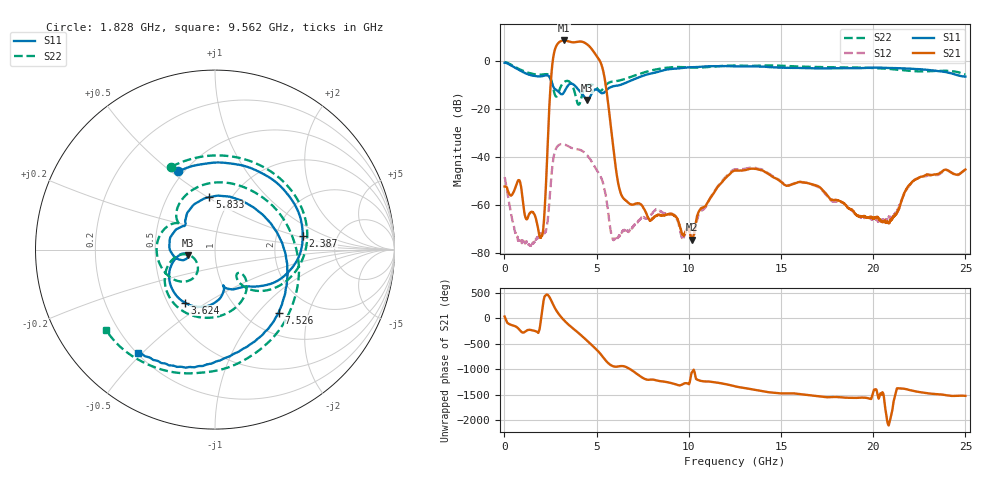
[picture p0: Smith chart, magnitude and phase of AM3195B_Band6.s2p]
!Agilent Technologies,E8364B,MY43040894,A.07.50.67
!Agilent E8364B: A.07.50.67
!Date: Wednesday, July 07, 2021 13:18:51
!Correction: S11(Full 2 Port(1,2))
!S21(Full 2 Port(1,2))
!S12(Full 2 Port(1,2))
!S22(Full 2 Port(1,2))
!S2P File: Measurements: S11, S21, S12, S22:
# Hz S  dB  R 50
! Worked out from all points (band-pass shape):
!   8001 points, 10 MHz to 25 GHz, reference 50 ohm
!   highest |S21| = 8.68 dB at 3.227 GHz (marker M1); lowest = -74.6 dB at 10.18 GHz (marker M2)
!   |S21| within 3 dB of the highest: 2.773 GHz to 4.672 GHz (1.899 GHz wide, 51 % of centre)
!   lowest |S11| = -16.2 dB at 4.489 GHz (marker M3), VSWR 1.37, Z = 36.8 - j2.45 ohm
!   |S11| at or under -10 dB: 2.614 GHz to 3.463 GHz (848.7 MHz wide, 27.9 % of centre); 3.792 GHz to 6.231 GHz (2.439 GHz wide, 48.7 % of centre)
!   |S22| runs from -18.2 to -0.3 dB; largest |S21 - S12| = 2.7
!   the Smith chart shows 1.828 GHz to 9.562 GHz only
!   S11 on the Smith chart (normalised r, x): 1.828 GHz: 0.47, +0.53; 2.387 GHz: 2.82, +0.58; 3.624 GHz: 0.61, -0.41; 5.833 GHz: 0.80, +0.51; 7.526 GHz: 1.39, -1.30; 9.562 GHz: 0.20, -0.48
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1e7  -0.62 -8.4  -52.36 38.5  -48.41 -7.3  -0.34 -9.1
1.828022e9  -6.34 115.3  -70.14 77.2  -73.52 154.5  -5.64 117.8
2.387174e9  -6.11 9.1  -26.60 90.3  -63.31 -63.2  -5.63 10.8
2.799509e9  -11.96 -57.7  6.15 165.7  -36.50 0.5  -14.78 -48.1
2.968191e9  -13.03 -74.1  7.94 76.5  -34.93 -86.6  -12.28 -44.6
3.227462e9  -13.03 -77.0  8.68 -33.6  -34.73 166.3  -8.79 -81.2
3.405516e9  -10.61 -90.0  8.46 -98.2  -35.29 103.9  -8.22 -110.6
3.624179e9  -9.37 -119.9  7.99 -168.2  -36.18 36.5  -9.40 -145.2
3.930306e9  -11.13 -155.4  8.07 100.9  -36.77 -50.2  -16.82 -167.3
4.177082e9  -13.29 -168.9  8.19 22.7  -37.30 -123.5  -15.03 -126.9
4.489458e9  -16.21 -167.9  7.04 -80.7  -39.32 141.1  -10.17 -158.3
4.726862e9  -13.56 -165.1  5.16 -161.4  -41.89 67.0  -9.76 176.4
4.979886e9  -11.76 165.8  2.44 111.3  -45.17 -11.8  -10.90 150.8
5.83267e9  -10.65 96.1  -31.25 147.6  -73.44 150.9  -8.54 89.7
7.525742e9  -6.03 -44.7  -61.11 -96.6  -65.19 -86.3  -4.77 -52.8
8.341041e9  -4.41 -83.1  -64.18 -148.5  -62.22 -151.5  -3.27 -94.5
9.562428e9  -2.88 -126.9  -70.17 125.2  -72.14 123.2  -2.44 -143.8
1.017781e10  -2.52 -145.9  -74.56 21.7  -74.25 -37.3  -2.65 -163.0
1.2505e10  -2.13 146.5  -45.69 102.4  -45.16 104.3  -1.80 131.5
1.667208e10  -2.93 21.5  -51.40 -78.3  -51.57 -80.5  -2.37 4.6
2.083604e10  -2.84 -69.6  -67.56 51.1  -65.20 101.2  -3.19 -82.9
2.5e10  -6.42 -119.7  -45.25 -85.7  -45.64 -81.3  -5.50 -131.5
